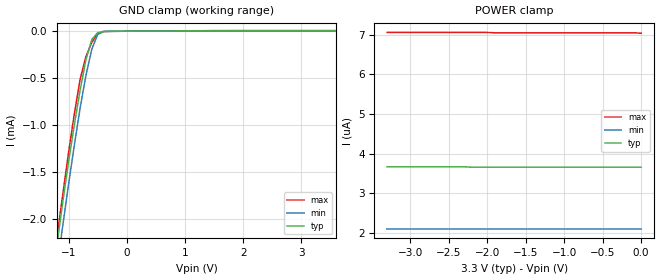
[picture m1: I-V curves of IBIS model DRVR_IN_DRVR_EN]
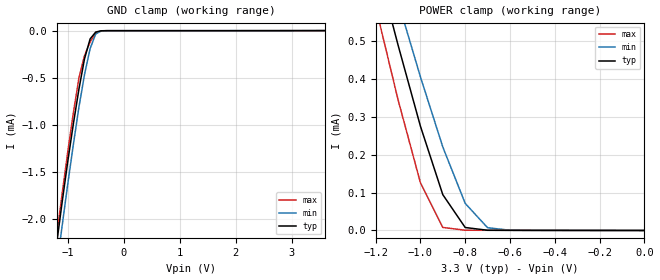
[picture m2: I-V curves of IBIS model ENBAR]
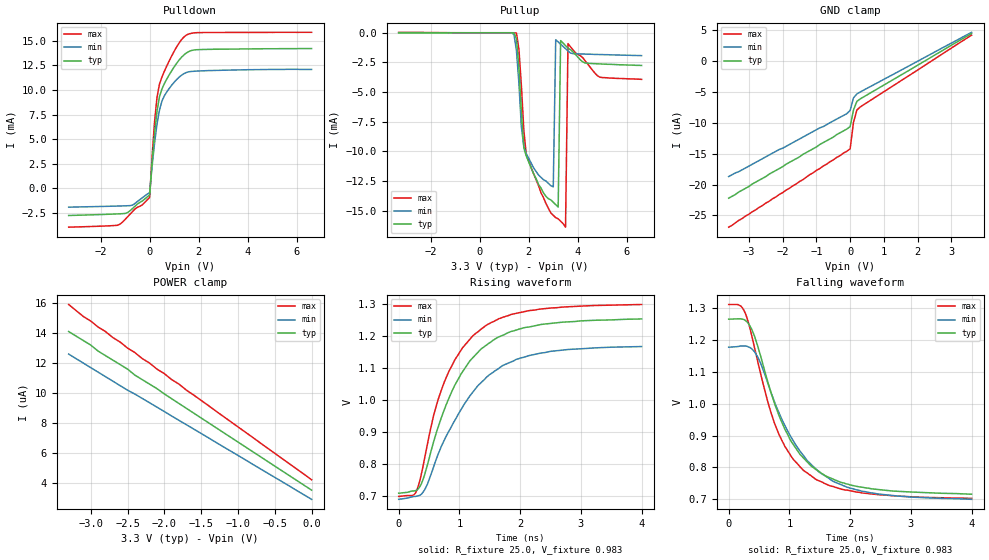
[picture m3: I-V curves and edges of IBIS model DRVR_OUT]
|   Texas Instruments Incorporated
|   Data Transmissions Products
|   IBIS Model for SN65MLVD047
|   16D SOIC Package
[IBIS Ver]   3.2
[Comment char]   |_char
[File name]   mlvd047d.ibs
[File Rev]   1.0
[Date]   3Feb04
[Source]   File originated at Texas Instruments Incorporated.
   Data Transmission Products Group. All data based on
   Simulation Measurements.
[Notes]
[Disclaimer]
(C) Copyright Texas Instruments Incorporated 2004
   All rights reserved
  Texas Instruments Incorporated hereby grants the user of this IBIS
model a non-exclusive, nontransferable license to use this IBIS model
under the following terms.  Before using this IBIS model, the user
should read this license.  If the user does not accept these terms,
the IBIS model should be returned to Texas Instruments within 30 days.
  The user is granted this license only to use the IBIS model and
is not granted rights to sell, load, rent, lease or license the IBIS
model in whole or in part, or in modified form to anyone other than
user.  User may modify the IBIS model to suit its specific applications
but rights to derivative works and such modifications shall belong to
Texas Instruments.
  This IBIS model is provided on an "AS IS" basis and Texas Instruments
makes absolutely no warranty with respect to the information contained
herein.  TEXAS INSTRUMENTS DISCLAIMS AND CUSTOMER WAIVES ALL WARRANTIES,
EXPRESS OR IMPLIED, INCLUDING WARRANTIES OF MERCHANTABILITY OR FITNESS
FOR A PARTICULAR PURPOSE. The entire risk as to quality and performance
is with the Customer. ACCORDINGLY, IN NO EVENT SHALL THE COMPANY BE LIABLE
FOR ANY DAMAGES, WHETHER IN CONTRACT OR TORT,INCLUDING ANY LOST PROFITS
OR OTHER INCIDENTAL, CONSEQUENTIAL, EXEMPLARY, OR PUNITIVE DAMAGES ARISING
OUT OF THE USE OR APPLICATION OF THE IBIS model provided in this package.
Further, Texas Instruments reserves the right to discontinue or make changes
without notice to any product herein to improve reliability, function, or
design. Texas Instruments does not convey any license under patent rights
or any other intellectual property rights, including those of third parties.
Contact Texas Instruments at ATTN:DATA TRANSMISSIONS
[Copyright]   Copyright 2004, Texas Instruments, All Rights Reserved
[Component]   SN65MLVD047
[Manufacturer]  Texas Instruments Incorporated
[Package]
|   typ   min   max
R_pkg   0.042   0.035   0.049
L_pkg   3.147nH   2.164nH   4.219nH
C_pkg   0.404pF   0.241pF   0.562pF
[Pin]   signal_name   model_name   R_pin   L_pin   C_pin
1   EN   DRVR_IN_DRVR_EN   0.049   4.215n   0.562p
2   1A   DRVR_IN_DRVR_EN   0.046   3.675n   0.480p
3   2A   DRVR_IN_DRVR_EN   0.037   2.527n   0.332p
4   VCC   POWER   0.035   2.164n   0.241p
5   GND   GND   0.035   2.164n   0.241p
6   3A   DRVR_IN_DRVR_EN   0.037   2.527n   0.332p
7   4A   DRVR_IN_DRVR_EN   0.046   3.675n   0.480p
8   ENBAR   ENBAR   0.049   4.215n   0.562p
9   4Z   DRVR_OUT   0.049   4.219n   0.562p
10   4Y   DRVR_OUT   0.046   3.679n   0.480p
11   3Y   DRVR_OUT   0.037   2.531n   0.333p
12   3Z   DRVR_OUT   0.035   2.168n   0.241p
13   2Z   DRVR_OUT   0.035   2.168n   0.241p
14   2Y   DRVR_OUT   0.037   2.531n   0.333p
15   1Y   DRVR_OUT   0.046   3.679n   0.480p
16   1Z   DRVR_OUT   0.049   4.219n   0.562p
| Models and submodels in the file (3): DRVR_IN_DRVR_EN (Input), ENBAR (Input), DRVR_OUT (3-state)
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|   Driver/Driver Enable Model
[Model]   DRVR_IN_DRVR_EN
Model_type   Input
|Signals   1D thru 8D, 1DE thru 8DE
Vinh = 2.0
Vinl = 0.8
|   typ   min   max
C_comp   4.04pF   3.87pF   4.24pF
|   typ   min   max
[Temperature Range]   25.0   -40   85
[Voltage range]   3.3V   3.0V   3.6V
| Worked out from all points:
|   GND clamp passes 1 mA (typ) near -0.90 V on its own axis
[GND_clamp]
|   Voltage   I(typ)   I(min)   I(max)
-3.6V     -16.3mA    -15.9mA    -16.8mA
-1.2V     -2.27mA    -2.53mA    -2.19mA
-1.1V     -1.82mA    -2.07mA    -1.74mA
-1V       -1.39mA    -1.63mA    -1.29mA
-900mV    -992uA     -1.21mA    -876uA
-800mV    -621uA     -813uA     -505uA
-700mV    -299uA     -466uA     -268uA
-600mV    -88.7uA    -191uA     -120uA
-500mV    -15.9uA    -35.6uA    -26.5uA
-400mV    -2.37uA    -3.13uA    -3.62uA
-300mV    -1.1uA     -793nA     -1.87uA
3.6V      3.66uA     2.11uA     7.04uA
[Power_clamp]
| Note that the[POWER_clamp]voltage table is referenced to Vcc
| and is calculated using Vtable=Vcc - Vmeasured.
|   Voltage   I(typ)   I(min)   I(max)
-3.3V     3.67uA     2.11uA     7.06uA
-2.3V     3.67uA     2.11uA     7.06uA
-2.2V     3.66uA     2.11uA     7.06uA
-2V       3.66uA     2.11uA     7.06uA
-1.9V     3.66uA     2.11uA     7.05uA
-100mV    3.66uA     2.11uA     7.05uA
0V        3.66uA     2.11uA     7.04uA
|   Enbar Model
[Model]   ENBAR
Model_type   Input
|Signals   ENBAR
Vinh = 2.0
Vinl = 0.8
|   typ   min   max
C_comp   5.94pF   5.59pF   7.01pF
|   typ   min   max
[Temperature Range]   25.0   -40   85
[Voltage range]   3.3V   3.0V   3.6V
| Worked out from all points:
|   GND clamp passes 1 mA (typ) near -0.90 V on its own axis
|   POWER clamp passes 1 mA (typ) near -1.32 V on its own axis
[GND_clamp]
|   Voltage   I(typ)   I(min)   I(max)
-3.6V     -16.3mA    -15.9mA    -16.8mA
-1.2V     -2.27mA    -2.53mA    -2.19mA
-1.1V     -1.82mA    -2.07mA    -1.73mA
-1V       -1.39mA    -1.63mA    -1.29mA
-900mV    -991uA     -1.21mA    -875uA
-800mV    -621uA     -812uA     -503uA
-700mV    -298uA     -465uA     -266uA
-600mV    -87.7uA    -190uA     -119uA
-500mV    -14.9uA    -34.9uA    -24.6uA
-400mV    -1.52uA    -2.61uA    -1.98uA
-300mV    -611nA     -513nA     -863nA
3.6V      162nA      569nA      64.5pA
[Power_clamp]
| Note that the[POWER_clamp]voltage table is referenced to Vcc
| and is calculated using Vtable=Vcc - Vmeasured.
|   Voltage   I(typ)   I(min)   I(max)
-3.3V     5.83mA     5.46mA     6.22mA
-1.2V     714uA      811uA      590uA
-1.1V     489uA      604uA      345uA
-1V       275uA      405uA      126uA
-900mV    94.4uA     220uA      8.03uA
-800mV    7.83uA     71.4uA     651nA
-700mV    564nA      7.25uA     518nA
-600mV    340nA      569nA      441nA
0V        64.2pA     82.8pA     64.5pA
|   Driver Output Model
[Model]   DRVR_OUT
Model_type   3-state
| Signals   1Y through 4Y, 1Z through 4Z
Vmeas = 1.0V   |Reference voltage for timing measurements
Cref = 3pF   |Timing specification test load capacitance value
| variable   typ   min   max
C_comp   3.93pF   3.71pF   4.23pF
|   typ   min   max
[Temperature Range]   25.0   -40   85
[Voltage range]   3.3V   3.0V   3.6V
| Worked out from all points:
|   slope of the pulldown table from 0 to 0.495 V, typ, clamps not added: 46.2 ohm
|   rising waveform, R_fixture 25.0, V_fixture 0.983: 20-80 % time 780ps typ, 884ps min, 694ps max; typ from 0.709 V to 1.25 V
|   falling waveform, R_fixture 25.0, V_fixture 0.983: 20-80 % time 734ps typ, 822ps min, 659ps max; typ from 1.26 V to 0.716 V
[Pulldown]
|   Voltage   I(typ)   I(min)   I(max)
-3.3V     -2.76mA    -1.912mA   -3.946mA
-1.3V     -2.598mA   -1.8mA     -3.75mA
-700mV    -2.055mA   -1.706mA   -2.366mA
0V        -661.3uA   -444.3uA   -917.6uA
100mV     2.646mA    2.245mA    3.252mA
200mV     5.55mA     4.605mA    6.771mA
300mV     7.851mA    6.536mA    9.257mA
400mV     9.314mA    7.951mA    10.59mA
700mV     11.12mA    9.812mA    12.45mA
1.4V      13.57mA    11.66mA    15.39mA
1.9V      14.09mA    11.92mA    15.82mA
6.6V      14.21mA    12.09mA    15.86mA
[Pullup]
|   Voltage   I(typ)   I(min)   I(max)
| Note that the[Pullup]voltage table is referenced to Vcc
| and is calculated using Vtable=Vcc - Vmeasured.
-3.3V     768nA      50nA       36.2uA
1.5V      -514uA     -1.5mA     -22.1uA
1.8V      -9.71mA    -9.57mA    -8.22mA
1.9V      -10.4mA    -10.2mA    -10.3mA
3V        -14.3mA    -13mA      -15.4mA
3.1V      -14.5mA    -590uA     -15.6mA
3.2V      -14.7mA    -775uA     -15.7mA
3.3V      -661uA     -965uA     -15.9mA
3.5V      -1.09mA    -1.34mA    -16.4mA
3.6V      -1.29mA    -1.54mA    -918uA
4.9V      -2.63mA    -1.84mA    -3.75mA
6.6V      -2.76mA    -1.93mA    -3.93mA
[GND_clamp]
|   Voltage   I(typ)   I(min)   I(max)
| Outputs in High Impedance (off)
-3.6V     -22.2uA    -18.7uA    -26.9uA
-800mV    -13.2uA    -10.6uA    -17uA
-100mV    -11uA      -8.51uA    -14.6uA
0V        -10.6uA    -7.97uA    -14.2uA
100mV     -7.89uA    -5.93uA    -9.89uA
200mV     -6.51uA    -5.3uA     -7.91uA
400mV     -5.78uA    -4.68uA    -7.05uA
3.6V      4.51uA     4.69uA     4.24uA
[Power_clamp]
| Note that the[POWER_clamp]voltage table is referenced to Vcc
| and is calculated using Vtable=Vcc - Vmeasured.
|   Voltage   I(typ)   I(min)   I(max)
-3.3V     14.1uA     12.6uA     15.9uA
-3.1V     13.5uA     12uA       15.1uA
-3V       13.2uA     11.7uA     14.8uA
-2.9V     12.8uA     11.4uA     14.4uA
-2.8V     12.5uA     11.1uA     14.1uA
-2.5V     11.6uA     10.2uA     13uA
-2.4V     11.2uA     9.94uA     12.7uA
-2.1V     10.3uA     9.07uA     11.6uA
-1.8V     9.31uA     8.19uA     10.6uA
-1.7V     8.99uA     7.9uA      10.2uA
0V        3.55uA     2.94uA     4.24uA
[Ramp]
|   typ   min   max
dV/dt_r   334mV/819ps   292mV/930ps   369mV/724ps
dV/dt_f   334mV/774ps   292mV/866ps   369mV/702ps
R_load = 25ohm  | Note: The measurement is single-ended with 25ohm
|   to common mode voltage.
[Rising Waveform]
R_fixture = 25.0
V_fixture = 0.983
V_fixture_min = 0.928
V_fixture_max = 0.999
C_fixture = 0p
L_fixture = 0n
|   V(typ)   V(min)   V(max)
0s        709mV      690mV      699mV
275ps     717mV      699mV      709mV
350ps     730mV      703mV      749mV
450ps     782mV      728mV      840mV
575ps     869mV      791mV      951mV
750ps     969mV      874mV      1.055V
1.025ns   1.08V      969mV      1.154V
1.375ns   1.161V     1.057V     1.223V
2.15ns    1.227V     1.138V     1.278V
4ns       1.252V     1.166V     1.297V
[Falling Waveform]
R_fixture = 25.0
V_fixture = 0.983
V_fixture_min = 0.928
V_fixture_max = 0.999
C_fixture = 0p
L_fixture = 0n
|   V(typ)   V(min)   V(max)
0s        1.265V     1.177V     1.311V
225ps     1.265V     1.181V     1.301V
425ps     1.212V     1.163V     1.176V
650ps     1.064V     1.061V     1.002V
825ps     965mV      973mV      905mV
1.025ns   883mV      896mV      836mV
1.25ns    826mV      833mV      788mV
1.725ns   763mV      756mV      740mV
2.2ns     738mV      725mV      720mV
4ns       716mV      700mV      703mV
